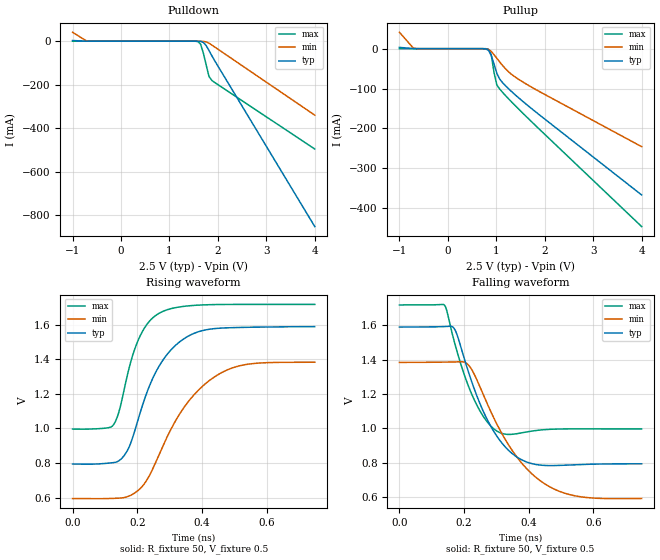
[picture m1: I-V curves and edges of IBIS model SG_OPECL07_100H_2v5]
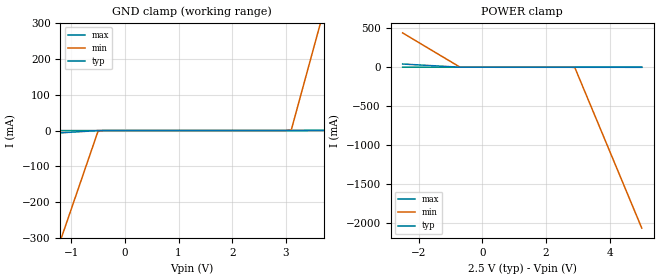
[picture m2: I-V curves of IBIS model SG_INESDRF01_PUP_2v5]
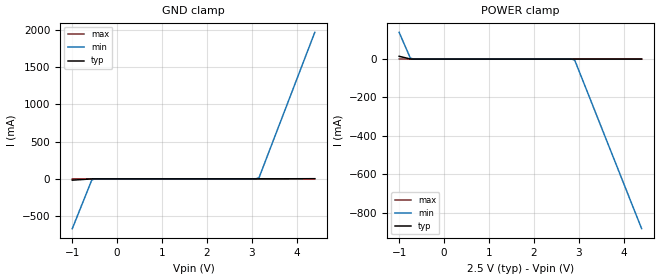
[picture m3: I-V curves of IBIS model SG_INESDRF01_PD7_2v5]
|   This file is an IBIS representation of the   |
|   Integrated Device Technology, Inc.   |
|   ICS853S011BI   |
|   LOW SKEW, 1-TO-2, DIFFERENTIAL-TO-2.5V,3.3V LVPECL/ECL FANOUT BUFFER   |
[IBIS Ver]   4.1
[File name]   853s011bi.ibs
[File Rev]   1.0
[Date]   26 May 2010
[Source]   Originated at Integrated Device Technology, Inc.
[Disclaimer]
IDT hereby grants the user of this IBIS model a non-exclusive,
nontransferable license to use this IBIS model under the following terms.
Before using this IBIS model, the user should read this license.
If the user does not accept these terms,  the IBIS model should be
returned to IDT within 30 days.
   The user is granted this license only to use the IBIS model and
is not granted rights to sell, load, rent, lease or license the IBIS
model in whole or in part, or in modified form to anyone other than
user. User may modify the IBIS model to suit its specific
applications but rights to derivative works and such modifications
shall belong to IDT.
   This IBIS model is provided on an "AS IS" basis and IDT makes
absolutely no warranty with respect to the information contained
herein. IDT DISCLAIMS AND CUSTOMER WAIVES ALL WARRANTIES, EXPRESS
OR IMPLIED, INCLUDING WARRANTIES OF MERCHANTABILITY OR FITNESS FOR
A PARTICULAR PURPOSE. The entire risk as to quality and performance
is with the Customer. ACCORDINGLY, IN NO EVENT SHALL THE COMPANY BE
LIABLE FOR ANY DAMAGES, WHETHER IN CONTRACT OR TORT,INCLUDING ANY
LOST PROFITS OR OTHER INCIDENTAL, CONSEQUENTIAL, EXEMPLARY, OR
PUNITIVE DAMAGES ARISING OUT OF THE USE OR APPLICATION OF THE IBIS
model provided in this package. Further, IDT reserves the right to
make changes without notice to any product herein to improve
reliability, function, or design. IDT does not convey any license
under patent rights or any other intellectual property rights,
including those of third parties.
   IDT is not obligated to provide maintenance or support
for the licensed IBIS model.
[Copyright]   Copyright 2010 by Integrated Device Technology, Inc.
[Component]   ICS853S011BMI
[Manufacturer] Integrated Device Technology, Inc.
[Package]
|SOIC 8 Lead
|   typ   min   max
R_pkg   57.05m   55.5m   58.6m
L_pkg   1.769nH   1.570nH   1.968nH
C_pkg   0.269pF   0.252pF   0.286pF
[Pin] signal_name   model_name   R_pin   L_pin   C_pin
1   Q0   SG_OPECL07_100H   58.6m   1.968n   0.286p
2   nQ0   SG_OPECL07_100H   55.5m   1.570n   0.252p
3   Q1   SG_OPECL07_100H   55.5m   1.570n   0.252p
4   nQ1   SG_OPECL07_100H   56.6m   1.968n   0.286p
5   VEE   GND   58.6m   1.968n   0.286p
6   nPCLK   SG_INESDRF01_PUP   55.5m   1.570n   0.252p
7   PCLK   SG_INESDRF01_PD7   55.5m   1.570n   0.252p
8   VCC   POWER   56.6m   1.968n   0.286p
[Diff Pin]  inv_pin  vdiff tdelay_typ tdelay_min  tdelay_max
1   2   NA   0  0  0
3   4   NA   0  0  0
7   6   0.15 0  0  0
[Component]   ICS853S011BGI
[Manufacturer] Integrated Device Technology, Inc.
[Package]
|TSSOP 8 Lead
|   typ   min   max
R_pkg   52.5m   48.8m   56.2m
L_pkg   1.381nH   1.275nH   1.486nH
C_pkg   0.236pF   0.230pF   0.242pF
[Pin] signal_name   model_name   R_pin   L_pin   C_pin
1   Q0   SG_OPECL07_100H   56.2m   1.486n   0.242p
2   nQ0   SG_OPECL07_100H   48.8m   1.275n   0.230p
3   Q1   SG_OPECL07_100H   48.8m   1.275n   0.230p
4   nQ1   SG_OPECL07_100H   56.2m   1.468n   0.242p
5   VEE   GND   56.2m   1.486n   0.242p
6   nPCLK   SG_INESDRF01_PUP   48.8m   1.275n   0.230p
7   PCLK   SG_INESDRF01_PD7   48.8m   1.275n   0.230p
8   VCC   POWER   56.2m   1.468n   0.242p
[Diff Pin]  inv_pin  vdiff tdelay_typ tdelay_min  tdelay_max
1   2   NA   0  0  0
3   4   NA   0  0  0
7   6   0.15 0  0  0
[Model Selector] SG_OPECL07_100H
SG_OPECL07_100H_2v5  Buffer selection for 2v5
SG_OPECL07_100H_3v3  Buffer selection for 3v3
[Model Selector] SG_INESDRF01_PUP
SG_INESDRF01_PUP_2v5  Buffer selection for 2v5
SG_INESDRF01_PUP_3v3  Buffer selection for 3v3
[Model Selector] SG_INESDRF01_PD7
SG_INESDRF01_PD7_2v5  Buffer selection for 2v5
SG_INESDRF01_PD7_3v3  Buffer selection for 3v3
| Models and submodels in the file (6): SG_OPECL07_100H_2v5 (Output_ECL), SG_INESDRF01_PUP_2v5 (Input), SG_INESDRF01_PD7_2v5 (Input), SG_OPECL07_100H_3v3 (Output_ECL), SG_INESDRF01_PUP_3v3 (Input), SG_INESDRF01_PD7_3v3 (Input)
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[Model] SG_OPECL07_100H_2v5
Model_type   Output_ECL
Polarity   Non-Inverting
|   typ   min   max
C_comp   2pF   1.5pF   2.5pF
Vmeas = 1.22V
Rref = 50
Cref = 0
Vref = 0.5V
|   typ   min   max
[Voltage range]   2.5V   2.375V   2.625V
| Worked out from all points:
|   rising waveform, R_fixture 50, V_fixture 0.5: 20-80 % time 106ps typ, 147ps min, 70.2ps max; typ from 0.794 V to 1.59 V
|   falling waveform, R_fixture 50, V_fixture 0.5: 20-80 % time 105ps typ, 149ps min, 77.6ps max; typ from 1.59 V to 0.794 V
[Pulldown]
|Voltage   I (typ)   I (min)   I (max)
-999mV    3.236mA    41.07mA    51.47uA
-711.7mV  75.61uA    1.458mA    617.8nA
-654.2mV  8.078uA    226.5uA    35.41nA
1.587V    -86.48uA   -19.21uA   -1.152mA
1.644V    -752.2uA   -118.1uA   -13.49mA
1.702V    -5.318mA   -685.4uA   -55.72mA
1.759V    -20.29mA   -3.152mA   -109.3mA
1.817V    -42.51mA   -9.053mA   -161.7mA
1.874V    -65.92mA   -17.23mA   -179.8mA
4V        -852mA     -339.8mA   -495.5mA
[Pullup]
|Voltage   I (typ)   I (min)   I (max)
-999mV    3.236mA    41.07mA    51.47uA
-711.7mV  75.61uA    1.458mA    617.8nA
724.8mV   -60.94uA   -68.32uA   -5.553uA
839.7mV   -4.039mA   -2.1mA     -1.493mA
897.2mV   -17.48mA   -7.16mA    -16.22mA
954.6mV   -39.41mA   -15.28mA   -60.59mA
1.012V    -62.14mA   -24.41mA   -91.49mA
1.07V     -76.16mA   -33.41mA   -101.1mA
1.127V    -84.99mA   -41.9mA    -109.3mA
1.357V    -112.3mA   -68.3mA    -138.8mA
1.702V    -147.8mA   -94.78mA   -180.2mA
4V        -367.2mA   -246mA     -446.5mA
[Ramp]
|   typ   min   max
dV/dt_r   0.636/0.167n   0.631/0.224n   0.577/0.112n
dV/dt_f   0.649/0.158n   0.638/0.221n   0.605/0.118n
R_load =   50.0000
[Rising Waveform]
R_fixture = 50
V_fixture = 0.5   | VCC_typ - 2V
V_fixture_max = 0.625   | VCC_max - 2V
V_fixture_min = 0.375   | VCC_min - 2V
C_fixture = 0.0p
| Time   typ   min   max
0s        794.1mV    594.5mV    996.6mV
120.9ps   801.1mV    594.9mV    1.011V
154.7ps   831.9mV    598.4mV    1.182V
177.9ps   906.2mV    611.4mV    1.371V
205ps     1.065V     644.6mV    1.519V
271.8ps   1.373V     866.2mV    1.671V
354.4ps   1.531V     1.146V     1.709V
453.5ps   1.58V      1.315V     1.718V
550.3ps   1.586V     1.374V     1.718V
749.2ps   1.589V     1.384V     1.718V
[Falling Waveform]
R_fixture = 50
V_fixture = 0.5   | VCC_typ - 2V
V_fixture_max = 0.625   | VCC_max - 2V
V_fixture_min = 0.375   | VCC_min - 2V
C_fixture = 0.0p
| Time   typ   min   max
0s        1.589V     1.384V     1.718V
138.1ps   1.593V     1.385V     1.719V
167.4ps   1.586V     1.386V     1.521V
219.2ps   1.295V     1.355V     1.218V
263.5ps   1.082V     1.178V     1.058V
306.3ps   940.9mV    1.007V     978.9mV
385.1ps   810.5mV    782.6mV    976.1mV
474.5ps   783.2mV    650.3mV    995.1mV
574.3ps   790.4mV    598.3mV    996.8mV
749.2ps   793.7mV    591.6mV    996.5mV
[Model] SG_INESDRF01_PUP_2v5
Model_type   Input
Polarity   Non-Inverting
Vinl = 0.7V
Vinh = 1.7V
|   typ   min   max
C_comp   2pF   1.5pF   2.5pF
|   typ   min   max
[Voltage range]   2.5V   2.375V   2.625V
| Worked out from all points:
|   GND clamp passes 1 mA (typ) near -0.60 V on its own axis
|   POWER clamp passes 1 mA (typ) near -0.74 V on its own axis
[GND_clamp]
|Voltage   I (typ)   I (min)   I (max)
-2.5V     -18.68mA   -877.1mA   -176.4uA
-1.2V     -6.595mA   -308.2mA   -105.3uA
-1.1V     -5.665mA   -264.4mA   -99.8uA
-500mV    -88.13uA   -1.852mA   -66.99uA
3V        68.88uA    161.5uA    62.36uA
3.1V      73.77uA    2.321mA    66.06uA
3.6V      328.3uA    277.5mA    84.54uA
3.7V      379.2uA    332.6mA    88.23uA
5V        1.041mA    1.048A     136.3uA
[Power_clamp]
|Voltage   I (typ)   I (min)   I (max)
-2.5V     41.65mA    441.8mA    1.036mA
-700mV    124.7uA    1.074mA    74.72uA
2.9V      -65.32uA   -4.078mA   -58.67uA
5V        -544.4uA   -2.07A     -136.3uA
[Model] SG_INESDRF01_PD7_2v5
Model_type   Input
Polarity   Non-Inverting
Vinl = 0.7V
Vinh = 1.7V
|   typ   min   max
C_comp   2pF   1.5pF   2.5pF
|   typ   min   max
[Voltage range]   2.5V   2.375V   2.625V
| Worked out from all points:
|   GND clamp passes 1 mA (typ) near -0.58 V on its own axis
|   POWER clamp passes 1 mA (typ) near -0.76 V on its own axis
[GND_clamp]
|Voltage   I (typ)   I (min)   I (max)
-999mV    -17.25mA   -669.4mA   -57.61uA
-564.6mV  -245.6uA   -14.47mA   -7.295uA
-502.5mV  -27.9uA    -1.943mA   -6.234uA
3.035V    40.09uA    312uA      37.56uA
3.159V    51.32uA    15.14mA    39.1uA
4.4V      2.038mA    1.969A     54.5uA
[Power_clamp]
|Voltage   I (typ)   I (min)   I (max)
-999mV    14.5mA     139mA      411.1uA
-750.8mV  388.8uA    5.212mA    46.1uA
-688.7mV  72.95uA    733.8uA    41.21uA
2.787V    -3.782uA   -107uA     -1.999uA
2.911V    -6.009uA   -5.663mA   -3.535uA
4.4V      -171.1uA   -883.8mA   -21.97uA
